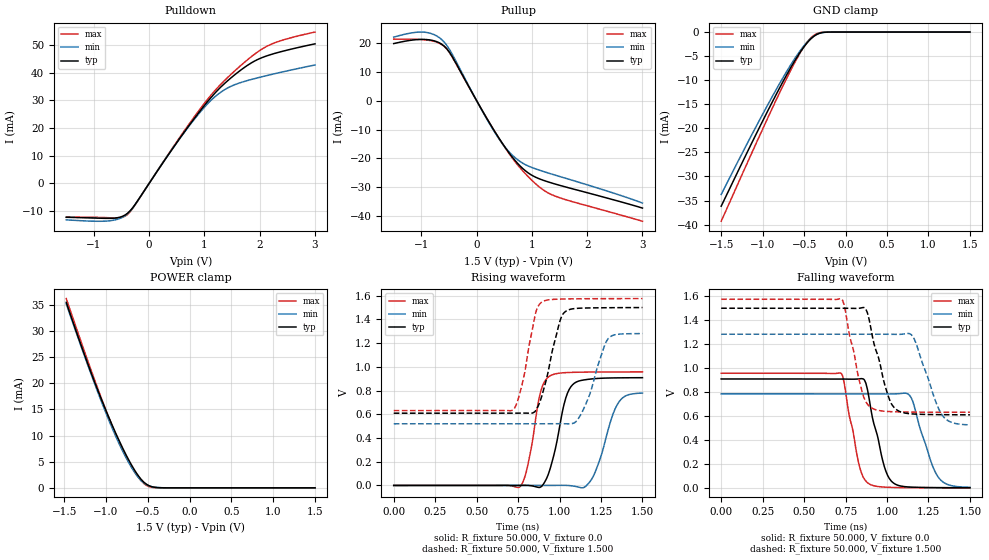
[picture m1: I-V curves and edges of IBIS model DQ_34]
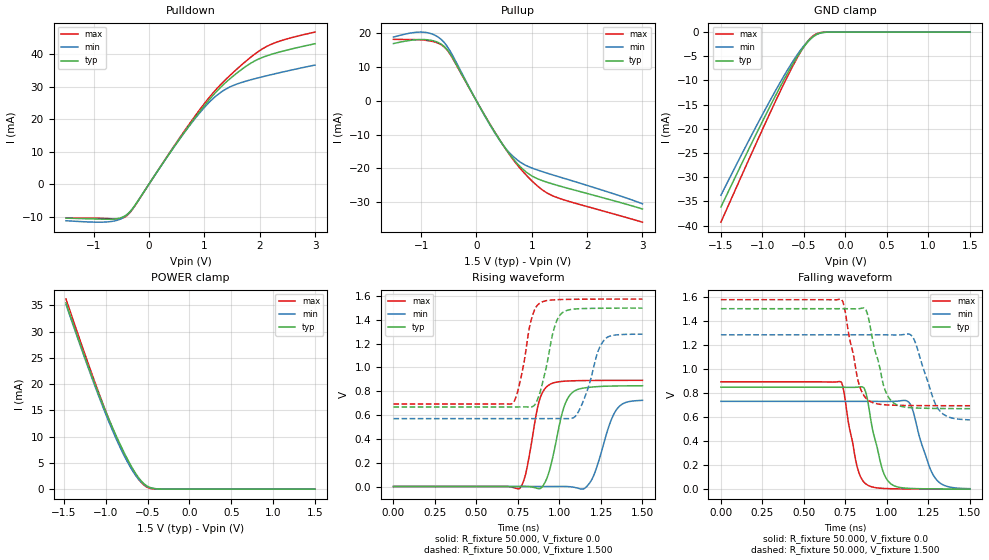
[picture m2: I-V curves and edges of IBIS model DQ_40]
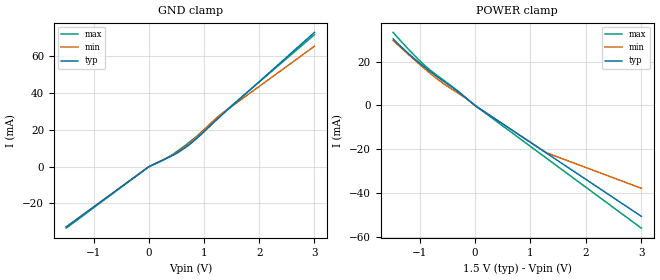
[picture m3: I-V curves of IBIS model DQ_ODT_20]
| This Model is valid for Temperature Range -40C<=Tc<=95C
| Valid for DDR3/DDR3L 1866 operation
| Part Number   VDD   VDDQ   Architecture   Package
| SCB13H8G162EF-11MI   1.35V/1.50V  1.35/1.50v  512Mx16   96-Ball BGA
[IBIS ver] 5.1
[File name] usslh8g16ei.ibs
[File Rev]  1.00
[Date]   2024-09-10
[Source]   Simulation of a silicon level SPICE model
[Notes]
   Date   Revision   Contents
   2024-09-10   1.00   Initial release
[Disclaimer]  The IBIS models are for modeling purpose only and are
   subject to change without any notice. UniIC is not
   responsible for any problems the models may cause.
[Copyright] Copyright 2024 UniIC Semiconductors Corp. All rights reserved
|   Component SCB13H8G162EF-11MI
[Component] SCB13H8G162EF-11MI
[Manufacturer] UniIC Semiconductors Corp.
[Package]
| variable   typ   min   max
R_pkg   1.088   0.726   1.603
L_pkg   2.210nH   1.650nH   4.223nH
C_pkg   1.078pF   0.834pF   1.397pF
[Pin]  signal_name   model_name   R_pin   L_pin   C_pin
A1   VDDQ   Power
A2   DQU5   DQ   1.194   2.482nH   0.989pF
A3   DQU7   DQ   1.212   2.596nH   0.995pF
A7   DQU4   DQ   1.136   2.498nH   0.908pF
A8   VDDQ   Power
A9   VSS   Gnd
B1   VSSQ   Gnd
B2   VDD   Power
B3   VSS   Gnd
B7   DQSUB   DQS   1.034   2.473nH   0.834pF
B8   DQU6   DQ   1.195   2.425nH   0.996pF
B9   VSSQ   Gnd
C1   VDDQ   Power
C2   DQU3   DQ   1.204   2.606nH   0.975pF
C3   DQU1   DQ   1.142   2.378nH   0.906pF
C7   DQSU   DQS   1.04   2.515nH   0.837pF
C8   DQU2   DQ   1.346   2.914nH   1.076pF
C9   VDDQ   Power
D1   VSSQ   Gnd
D2   VDDQ   Power
D3   DMU   DM   1.139   2.526nH   0.869pF
D7   DQU0   DQ   1.212   2.515nH   0.989pF
D8   VSSQ   Gnd
D9   VDD   Power
E1   VSS   Gnd
E2   VSSQ   Gnd
E3   DQL0   DQ   1.088   2.210nH   1.078pF
E7   DML   DM   1.142   2.270nH   1.071pF
E8   VSSQ   Gnd
E9   VDDQ   Power
F1   VDDQ   Power
F2   DQL2   DQ   1.179   2.247nH   1.161pF
F3   DQSL   DQS   0.879   1.897nH   0.875pF
F7   DQL1   DQ   1.107   2.286nH   1.067pF
F8   DQL3   DQ   1.097   2.267nH   1.062pF
F9   VSSQ   Gnd
G1   VSSQ   Gnd
G2   DQL6   DQ   1.169   2.247nH   1.239pF
G3   DQSLB   DQS   0.89   1.927nH   0.867pF
G7   VDD   Power
G8   VSS   Gnd
G9   VSSQ   Gnd
H1   VREFDQ   Power   1.041   2.295nH   1.271pF
H2   VDDQ   Power
H3   DQL4   DQ   1.08   2.278nH   1.098pF
H7   DQL7   DQ   1.107   2.255nH   1.078pF
H8   DQL5   DQ   1.099   2.285nH   1.058pF
H9   VDDQ   Power
J1   NC   NC
J2   VSS   Gnd
J3   RASB   CA   0.965   1.900nH   0.920pF
J7   CK   CK   1.222   2.820nH   1.098pF
J8   VSS   Gnd
J9   NC   NC
K1   ODT   CA   1.603   3.808nH   1.397pF
K2   VDD   Power
K3   CASB   CA   1.118   2.573nH   1.037pF
K7   CKB   CK   1.193   2.809nH   1.078pF
K8   VDD   Power
K9   CKE   CA   1.243   3.102nH   1.097pF
L1   NC   NC
L2   CSB   CA   1.42   3.871nH   1.155pF
L3   WEB   CA   0.976   2.017nH   0.917pF
L7   A10   CA   1.196   2.906nH   1.068pF
L8   ZQ   NC   0.958   2.238nH   1.063pF
L9   NC   NC
M1   VSS   Gnd
M2   BA0   CA   1.28   2.569nH   1.180pF
M3   BA2   CA   1.293   3.106nH   1.079pF
M7   A15   CA   1.351   3.042nH   1.202pF
M8   VREFCA   Power   0.726   1.650nH   0.861pF
M9   VSS   Gnd
N1   VDD   Power
N2   A3   CA   1.238   3.355nH   1.076pF
N3   A0   CA   1.097   3.149nH   0.979pF
N7   A12   CA   1.046   2.533nH   0.972pF
N8   BA1   CA   1.175   2.792nH   1.034pF
N9   VDD   Power
P1   VSS   Gnd
P2   A5   CA   1.211   3.936nH   0.963pF
P3   A2   CA   1.136   3.857nH   0.923pF
P7   A1   CA   1.016   2.953nH   0.869pF
P8   A4   CA   1.022   2.783nH   0.937pF
P9   VSS   Gnd
R1   VDD   Power
R2   A7   CA   1.265   4.223nH   1.016pF
R3   A9   CA   1.243   4.199nH   1.004pF
R7   A11   CA   1.152   3.663nH   0.954pF
R8   A6   CA   1.222   3.809nH   1.017pF
R9   VDD   Power
T1   VSS   Gnd
T2   RESETB   RST   1.573   3.493nH   1.305pF
T3   A13   CA   1.319   3.992nH   1.086pF
T7   A14   CA   1.172   3.553nH   1.018pF
T8   A8   CA   1.124   3.338nH   0.992pF
T9   VSS   Gnd
[Pin Mapping]  pulldown_ref   pullup_ref   gnd_clamp_ref   power_clamp_ref   ext_ref
A1   NC   VDDQ   NC   NC
A2   VSS   VDDQ   VSS   VDDQ
A3   VSS   VDDQ   VSS   VDDQ
A7   VSS   VDDQ   VSS   VDDQ
A8   NC   VDDQ   NC   NC
A9   VSS   NC   NC   NC
B1   VSSQ   NC   NC   NC
B2   NC   VDD   NC   NC
B3   VSS   NC   NC   NC
B7   VSS   VDDQ   VSS   VDDQ
B8   VSS   VDDQ   VSS   VDDQ
B9   VSSQ   NC   NC   NC
C1   NC   VDDQ   NC   NC
C2   VSS   VDDQ   VSS   VDDQ
C3   VSS   VDDQ   VSS   VDDQ
C7   VSS   VDDQ   VSS   VDDQ
C8   VSS   VDDQ   VSS   VDDQ
C9   NC   VDDQ   NC   NC
D1   VSSQ   NC   NC   NC
D2   NC   VDDQ   NC   NC
D3   VSS   VDDQ   VSS   VDDQ
D7   VSS   VDDQ   VSS   VDDQ
D8   VSSQ   NC   NC   NC
D9   NC   VDD   NC   NC
E1   VSS   NC   NC   NC
E2   VSSQ   NC   NC   NC
E3   VSS   VDDQ   VSS   VDDQ
E7   VSS   VDDQ   VSS   VDDQ
E8   VSSQ   NC   NC   NC
E9   NC   VDDQ   NC   NC
F1   NC   VDDQ   NC   NC
F2   VSS   VDDQ   VSS   VDDQ
F3   VSS   VDDQ   VSS   VDDQ
F7   VSS   VDDQ   VSS   VDDQ
F8   VSS   VDDQ   VSS   VDDQ
F9   VSSQ   NC   NC   NC
G1   VSSQ   NC   NC   NC
G2   VSS   VDDQ   VSS   VDDQ
G3   VSS   VDDQ   VSS   VDDQ
G7   NC   VDD   NC   NC
G8   VSS   NC   NC   NC
G9   VSSQ   NC   NC   NC
H1   NC   VREFDQ   NC   NC
H2   NC   VDDQ   NC   NC
H3   VSS   VDDQ   VSS   VDDQ
H7   VSS   VDDQ   VSS   VDDQ
H8   VSS   VDDQ   VSS   VDDQ
H9   NC   VDDQ   NC   NC
J1   NC   NC   NC   NC
J2   VSS   NC   NC   NC
J3   NC   NC   VSS   VDD
J7   NC   NC   VSS   VDD
J8   VSS   NC   NC   NC
J9   NC   NC   NC   NC
K1   NC   NC   VSS   VDD
K2   NC   VDD   NC   NC
K3   NC   NC   VSS   VDD
K7   NC   NC   VSS   VDD
K8   NC   VDD   NC   NC
K9   NC   NC   VSS   VDD
L1   NC   NC   NC   NC
L2   NC   NC   VSS   VDD
L3   NC   NC   VSS   VDD
L7   NC   NC   VSS   VDD
L8   NC   NC   NC   NC
L9   NC   NC   NC   NC
M1   VSS   NC   NC   NC
M2   NC   NC   VSS   VDD
M3   NC   NC   VSS   VDD
M7   NC   NC   VSS   VDD
M8   NC   VREFCA   NC   NC
M9   VSS   NC   NC   NC
N1   NC   VDD   NC   NC
N2   NC   NC   VSS   VDD
N3   NC   NC   VSS   VDD
N7   NC   NC   VSS   VDD
N8   NC   NC   VSS   VDD
N9   NC   VDD   NC   NC
P1   VSS   NC   NC   NC
P2   NC   NC   VSS   VDD
P3   NC   NC   VSS   VDD
P7   NC   NC   VSS   VDD
P8   NC   NC   VSS   VDD
P9   VSS   NC   NC   NC
R1   NC   VDD   NC   NC
R2   NC   NC   VSS   VDD
R3   NC   NC   VSS   VDD
R7   NC   NC   VSS   VDD
R8   NC   NC   VSS   VDD
R9   NC   VDD   NC   NC
T1   VSS   NC   NC   NC
T2   NC   NC   VSS   VDD
T3   NC   NC   VSS   VDD
T7   NC   NC   VSS   VDD
T8   NC   NC   VSS   VDD
T9   VSS   NC   NC   NC
[Diff pin]  inv_pin  vdiff   tdelay_typ   tdelay_min   tdelay_max
J7   K7   0.35   NA   NA   0
C7   B7   0.35   NA   NA   0
F3   G3   0.35   NA   NA   0
[Model Selector] DQ
DQ_34 34 Ohm Data I/O with no ODT
DQ_40 40 Ohm Data I/O with no ODT
DQ_ODT_20 Data Input with 20 Ohm ODT
DQ_ODT_30 Data Input with 30 Ohm ODT
DQ_ODT_40 Data Input with 40 Ohm ODT
DQ_ODT_60 Data Input with 60 Ohm ODT
DQ_ODT_120 Data Input with 120 Ohm ODT
[Model Selector] DQS
DQS_34 34 Ohm Data I/O with no ODT
DQS_40 40 Ohm Data I/O with no ODT
DQS_ODT_20 Data Strobe Input with 20 Ohm ODT
DQS_ODT_30 Data Strobe Input with 30 Ohm ODT
DQS_ODT_40 Data Strobe Input with 40 Ohm ODT
DQS_ODT_60 Data Strobe Input with 60 Ohm ODT
DQS_ODT_120 Data Strobe Input with 120 Ohm ODT
[Model Selector] DM
DQ_34 34 Ohm Data I/O with no ODT
DQ_40 40 Ohm Data I/O with no ODT
DQ_ODT_20 Data Input with 20 Ohm ODT
DQ_ODT_30 Data Input with 30 Ohm ODT
DQ_ODT_40 Data Input with 40 Ohm ODT
DQ_ODT_60 Data Input with 60 Ohm ODT
DQ_ODT_120 Data Input with 120 Ohm ODT
| Models and submodels in the file (17): DQ_34 (I/O), DQ_40 (I/O), DQ_ODT_20 (Input), DQ_ODT_30 (Input), DQ_ODT_40 (Input), DQ_ODT_60 (Input), DQ_ODT_120 (Input), DQS_34 (I/O), DQS_40 (I/O), DQS_ODT_20 (Input), DQS_ODT_30 (Input), DQS_ODT_40 (Input), DQS_ODT_60 (Input), DQS_ODT_120 (Input), CA (Input), CK (Input), RST (Input)
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|   Model DQ_34
[Model] DQ_34
Model_type I/O
Polarity   Non-Inverting
Enable   Active-High
Vinl =  0.615V
Vinh =  0.885V
Vmeas =  0.750V
Rref =  25.000
Vref =  0.750V
C_comp   0.989pF   0.937pF   1.002pF
C_comp_pullup   0.649pF   0.594pF   0.657pF
C_comp_pulldown   0.344pF   0.340pF   0.345pF
[Model Spec]
Vinh   0.885V   0.776V   0.922V
Vinl   0.615V   0.506V   0.652V
Vmeas   0.750V   0.641V   0.787V
Vref   0.750V   0.641V   0.787V
Rref   25.000   25.000   25.000
[Temperature Range]   45.000   95.000   -40.000
[Voltage Range]   1.500V   1.283V   1.575V
[C Comp Corner]
C_comp_pullup   0.657pF   0.594pF   0.649pF
C_comp_pulldown   0.345pF   0.344pF   0.340pF
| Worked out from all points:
|   slope of the pulldown table from 0 to 0.225 V, typ, clamps not added: 33.4 ohm
|   slope of the pullup table from 0 to 0.225 V, typ, clamps not added: 30.2 ohm
|   GND clamp passes 1 mA (typ) near -0.39 V on its own axis
|   POWER clamp passes 1 mA (typ) near -0.54 V on its own axis
|   rising waveform, R_fixture 50.000, V_fixture 0.0: 20-80 % time 84ps typ, 102ps min, 70.1ps max; typ from 0 V to 0.908 V
|   rising waveform, R_fixture 50.000, V_fixture 1.500: 20-80 % time 90.4ps typ, 105ps min, 77.3ps max; typ from 0.609 V to 1.5 V
|   falling waveform, R_fixture 50.000, V_fixture 0.0: 20-80 % time 88.6ps typ, 107ps min, 77.8ps max; typ from 0.909 V to 0.001 V
|   falling waveform, R_fixture 50.000, V_fixture 1.500: 20-80 % time 98.5ps typ, 113ps min, 86.9ps max; typ from 1.5 V to 0.61 V
[Pulldown]
|Voltage   I(typ)   I(min)   I(max)
-1.5V     -12.3mA    -13.23mA   -12.25mA
-718mV    -12.68mA   -13.57mA   -12.47mA
-534mV    -12.28mA   -12.74mA   -12.5mA
-396mV    -10.91mA   -11.08mA   -11.33mA
-258mV    -7.75mA    -7.81mA    -7.928mA
662mV     19.29mA    19.16mA    19.76mA
984mV     27.81mA    27.2mA     28.56mA
1.214V    33.18mA    31.75mA    34.12mA
1.674V    41.24mA    36.59mA    42.95mA
2.088V    45.86mA    38.81mA    49.17mA
2.41V     47.79mA    40.32mA    51.82mA
3V        50.5mA     42.84mA    54.76mA
[Pullup]
|Voltage   I(typ)   I(min)   I(max)
-1.5V     19.78mA    22.01mA    21.32mA
-956mV    21.22mA    23.74mA    21.11mA
-772mV    20.75mA    22.9mA     20.57mA
-588mV    18.92mA    20.32mA    18.82mA
-450mV    15.53mA    16.38mA    15.38mA
148mV     -4.96mA    -5.153mA   -4.926mA
470mV     -14.9mA    -14.99mA   -14.99mA
654mV     -19.76mA   -19.02mA   -20.09mA
838mV     -23.56mA   -21.7mA    -24.38mA
1.16V     -27.25mA   -24.21mA   -30.27mA
1.528V    -29.45mA   -26.4mA    -33.78mA
3V        -37.19mA   -35.46mA   -41.76mA
[GND_clamp]
|Voltage   I(typ)   I(min)   I(max)
-1.5V     -36.19mA   -33.76mA   -39.32mA
-1.066V   -20.77mA   -19.21mA   -22.66mA
-880mV    -14.41mA   -13.29mA   -15.7mA
-725mV    -9.363mA   -8.618mA   -10.11mA
-601mV    -5.649mA   -5.206mA   -5.957mA
-508mV    -3.226mA   -2.993mA   -3.205mA
-446mV    -1.897mA   -1.781mA   -1.722mA
-384mV    -901.4uA   -865.9uA   -696.2uA
-291mV    -146.4uA   -155.4uA   -72.34uA
-198mV    -7.512uA   -11.26uA   -1.231uA
1.5V      0A         0A         0A
[POWER_clamp]
|Voltage   I(typ)   I(min)   I(max)
-1.476V   35.46mA    35.16mA    36.18mA
-1.321V   28.28mA    28.05mA    28.95mA
-1.166V   21.46mA    21.17mA    21.92mA
-1.042V   16.37mA    15.95mA    16.55mA
-918mV    11.66mA    11.09mA    11.53mA
-794mV    7.371mA    6.793mA    7.041mA
-701mV    4.524mA    4.045mA    4.179mA
-608mV    2.178mA    1.886mA    1.878mA
-546mV    1.057mA    913.8uA    793uA
-453mV    217.8uA    210.4uA    93.91uA
-360mV    28.82uA    35.6uA     5.575uA
1.5V      0A         0A         0A
[Ramp]
| variable   typ   min   max
dV/dt_r   0.545/84.699p   0.467/0.102n   0.574/70.583p
dV/dt_f   0.534/98.035p   0.454/0.115n   0.566/87.057p
R_load = 50.000
[Rising Waveform]
R_fixture= 50.000
V_fixture= 0.0
V_fixture_min= 0.0
V_fixture_max= 0.0
|time   V(typ)   V(min)   V(max)
0s        737.6nV    1.747uV    141.1nV
759ps     462.8uV    155.3uV    -14.93mV
807ps     477.5uV    183uV      161.3mV
885ps     -13.67mV   123.7uV    785.7mV
947ps     159.5mV    199.3uV    927mV
1.048ns   779.1mV    -17.91uV   951.8mV
1.146ns   889.2mV    -17.46mV   955.1mV
1.215ns   900.5mV    113.7mV    956mV
1.349ns   906.8mV    683.7mV    956.8mV
1.5ns     908.3mV    778.9mV    957mV
[Rising Waveform]
R_fixture= 50.000
V_fixture= 1.500
V_fixture_min= 1.283
V_fixture_max= 1.575
|time   V(typ)   V(min)   V(max)
0s        609mV      519.8mV    631mV
719ps     609.2mV    519.9mV    635.2mV
772ps     609.7mV    520mV      839mV
840ps     611.8mV    520mV      1.344V
889ps     736mV      519.9mV    1.542V
1.009ns   1.413V     520.3mV    1.571V
1.087ns   1.49V      526.2mV    1.573V
1.174ns   1.496V     738.7mV    1.574V
1.294ns   1.498V     1.239V     1.575V
1.5ns     1.499V     1.28V      1.575V
[Falling Waveform]
R_fixture= 50.000
V_fixture= 0.0
V_fixture_min= 0.0
V_fixture_max= 0.0
|time   V(typ)   V(min)   V(max)
0s        909.2mV    785.1mV    957.1mV
723ps     908.6mV    784.7mV    957.7mV
828ps     909.7mV    784.7mV    212.8mV
858ps     908.7mV    784.7mV    85.99mV
994ps     135.6mV    784.1mV    5.604mV
1.04ns    39.2mV     784.5mV    3.459mV
1.125ns   7.984mV    785.3mV    1.663mV
1.155ns   5.781mV    723.1mV    1.314mV
1.304ns   2.119mV    99.51mV    457.8uV
1.5ns     756.2uV    4.492mV    159uV
[Falling Waveform]
R_fixture= 50.000
V_fixture= 1.500
V_fixture_min= 1.283
V_fixture_max= 1.575
|time   V(typ)   V(min)   V(max)
0s        1.5V       1.283V     1.575V
723ps     1.5V       1.283V     1.58V
741ps     1.5V       1.283V     1.531V
823ps     1.499V     1.283V     955.7mV
864ps     1.504V     1.283V     743.4mV
1.016ns   733.5mV    1.282V     637mV
1.134ns   619.8mV    1.288V     633mV
1.174ns   615.8mV    1.21V      632.4mV
1.334ns   611.2mV    604.1mV    631.5mV
1.5ns     609.9mV    525.6mV    631.2mV
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|   Model DQ_40
[Model] DQ_40
Model_type I/O
Polarity   Non-Inverting
Enable   Active-High
Vinl =  0.615V
Vinh =  0.885V
Vmeas =  0.750V
Rref =  25.000
Vref =  0.750V
C_comp   1.009pF   0.968pF   1.021pF
C_comp_pullup   0.661pF   0.619pF   0.670pF
C_comp_pulldown   0.349pF   0.347pF   0.351pF
[Model Spec]
Vinh   0.885V   0.776V   0.922V
Vinl   0.615V   0.506V   0.652V
Vmeas   0.750V   0.641V   0.787V
Vref   0.750V   0.641V   0.787V
Rref   25.000   25.000   25.000
[Temperature Range]   45.000   95.000   -40.000
[Voltage Range]   1.500V   1.283V   1.575V
[C Comp Corner]
C_comp_pullup   0.670pF   0.619pF   0.661pF
C_comp_pulldown   0.351pF   0.349pF   0.347pF
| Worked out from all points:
|   slope of the pulldown table from 0 to 0.225 V, typ, clamps not added: 39 ohm
|   slope of the pullup table from 0 to 0.225 V, typ, clamps not added: 35.1 ohm
|   GND clamp passes 1 mA (typ) near -0.39 V on its own axis
|   POWER clamp passes 1 mA (typ) near -0.54 V on its own axis
|   rising waveform, R_fixture 50.000, V_fixture 0.0: 20-80 % time 83ps typ, 97.7ps min, 69.3ps max; typ from 0 V to 0.846 V
|   rising waveform, R_fixture 50.000, V_fixture 1.500: 20-80 % time 77.4ps typ, 91.2ps min, 69.2ps max; typ from 0.668 V to 1.5 V
|   falling waveform, R_fixture 50.000, V_fixture 0.0: 20-80 % time 80.2ps typ, 97.4ps min, 70.6ps max; typ from 0.848 V to 0.001 V
|   falling waveform, R_fixture 50.000, V_fixture 1.500: 20-80 % time 84.3ps typ, 99.9ps min, 75.1ps max; typ from 1.5 V to 0.669 V
[Pulldown]
|Voltage   I(typ)   I(min)   I(max)
-1.5V     -10.47mA   -11.25mA   -10.41mA
-718mV    -10.8mA    -11.56mA   -10.62mA
-534mV    -10.48mA   -10.87mA   -10.65mA
-396mV    -9.313mA   -9.46mA    -9.664mA
-258mV    -6.621mA   -6.675mA   -6.77mA
708mV     17.57mA    17.43mA    17.99mA
984mV     23.77mA    23.26mA    24.39mA
1.214V    28.37mA    27.14mA    29.14mA
1.674V    35.27mA    31.27mA    36.68mA
2.088V    39.21mA    33.17mA    41.98mA
2.41V     40.86mA    34.46mA    44.24mA
3V        43.17mA    36.61mA    46.75mA
[Pullup]
|Voltage   I(typ)   I(min)   I(max)
-1.5V     17.01mA    18.93mA    18.26mA
-956mV    18.2mA     20.38mA    18.03mA
-772mV    17.79mA    19.65mA    17.55mA
-588mV    16.23mA    17.43mA    16.08mA
-450mV    13.33mA    14.06mA    13.15mA
194mV     -5.546mA   -5.745mA   -5.5mA
516mV     -13.91mA   -13.87mA   -13.99mA
838mV     -20.27mA   -18.65mA   -20.93mA
1.022V    -22.45mA   -20.04mA   -24.05mA
1.206V    -23.75mA   -21.07mA   -26.59mA
1.574V    -25.59mA   -22.94mA   -29.33mA
3V        -32.07mA   -30.53mA   -35.99mA
[GND_clamp]
|Voltage   I(typ)   I(min)   I(max)
-1.5V     -36.19mA   -33.76mA   -39.32mA
-1.066V   -20.77mA   -19.21mA   -22.66mA
-880mV    -14.41mA   -13.29mA   -15.7mA
-725mV    -9.363mA   -8.618mA   -10.11mA
-601mV    -5.649mA   -5.206mA   -5.957mA
-508mV    -3.226mA   -2.993mA   -3.205mA
-446mV    -1.897mA   -1.781mA   -1.722mA
-384mV    -901.4uA   -865.9uA   -696.2uA
-291mV    -146.4uA   -155.4uA   -72.34uA
-198mV    -7.512uA   -11.26uA   -1.231uA
1.5V      0A         0A         0A
[POWER_clamp]
|Voltage   I(typ)   I(min)   I(max)
-1.476V   35.46mA    35.16mA    36.18mA
-1.321V   28.28mA    28.05mA    28.95mA
-1.166V   21.46mA    21.17mA    21.92mA
-1.042V   16.37mA    15.95mA    16.55mA
-918mV    11.66mA    11.09mA    11.53mA
-794mV    7.371mA    6.793mA    7.041mA
-701mV    4.524mA    4.045mA    4.179mA
-608mV    2.178mA    1.886mA    1.878mA
-546mV    1.057mA    913.8uA    793uA
-453mV    217.8uA    210.4uA    93.91uA
-360mV    28.82uA    35.6uA     5.575uA
1.5V      0A         0A         0A
[Ramp]
| variable   typ   min   max
dV/dt_r   0.508/84.324p   0.434/99.318p   0.535/69.976p
dV/dt_f   0.499/84.534p   0.424/0.103n   0.529/75.094p
R_load = 50.000
[Rising Waveform]
R_fixture= 50.000
V_fixture= 0.0
V_fixture_min= 0.0
V_fixture_max= 0.0
|time   V(typ)   V(min)   V(max)
0s        786nV      1.889uV    135.1nV
760ps     330.3uV    105.6uV    -16.46mV
797ps     753.5uV    112.8uV    108.2mV
883ps     -17.55mV   66.45uV    740.1mV
933ps     102.6mV    52.74uV    849.8mV
1.04ns    713.7mV    345.1uV    885.8mV
1.145ns   827.2mV    -20.32mV   890.1mV
1.204ns   836.5mV    84.66mV    891mV
1.344ns   844.8mV    647.1mV    891.9mV
1.5ns     846.5mV    724mV      892.2mV
[Rising Waveform]
R_fixture= 50.000
V_fixture= 1.500
V_fixture_min= 1.283
V_fixture_max= 1.575
|time   V(typ)   V(min)   V(max)
0s        668.2mV    570.5mV    693.3mV
713ps     668.3mV    570.6mV    694.9mV
760ps     668.6mV    570.6mV    865.2mV
843ps     675.4mV    570.6mV    1.459V
885ps     800.6mV    570.6mV    1.544V
980ps     1.379V     570.9mV    1.569V
1.076ns   1.489V     573.7mV    1.573V
1.135ns   1.495V     689.5mV    1.574V
1.273ns   1.498V     1.237V     1.575V
1.5ns     1.499V     1.28V      1.575V
[Falling Waveform]
R_fixture= 50.000
V_fixture= 0.0
V_fixture_min= 0.0
V_fixture_max= 0.0
|time   V(typ)   V(min)   V(max)
0s        847.6mV    730.1mV    892.5mV
723ps     847.1mV    729.8mV    892.2mV
820ps     847.6mV    729.8mV    189.7mV
859ps     844.8mV    729.8mV    62.86mV
985ps     118.4mV    729mV      5.961mV
1.122ns   7.734mV    732.9mV    1.668mV
1.152ns   5.727mV    672.5mV    1.319mV
1.211ns   3.645mV    367.7mV    850.1uV
1.292ns   2.237mV    90.02mV    488.4uV
1.5ns     751.8uV    4.26mV     158.7uV
[Falling Waveform]
R_fixture= 50.000
V_fixture= 1.500
V_fixture_min= 1.283
V_fixture_max= 1.575
|time   V(typ)   V(min)   V(max)
0s        1.5V       1.283V     1.575V
725ps     1.5V       1.283V     1.579V
744ps     1.5V       1.283V     1.511V
827ps     1.499V     1.283V     895.9mV
864ps     1.505V     1.283V     773mV
998ps     793.6mV    1.283V     700.5mV
1.132ns   678.6mV    1.29V      695.3mV
1.172ns   675mV      1.215V     694.7mV
1.311ns   670.8mV    663.5mV    693.8mV
1.5ns     669.1mV    576.1mV    693.5mV
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|   Model DQ_ODT_20
[Model] DQ_ODT_20
Model_type Input
Polarity   Non-Inverting
Enable   Active-High
Vinl =  0.615V
Vinh =  0.885V
C_comp   0.913pF   0.802pF   0.924pF
C_comp_power_clamp   0.588pF   0.463pF   0.591pF
C_comp_gnd_clamp   0.336pF   0.322pF   0.338pF
[Model Spec]
Vinh   0.885V   0.776V   0.922V
Vinl   0.615V   0.506V   0.652V
[Temperature Range]   45.000   95.000   -40.000
[Voltage Range]   1.500V   1.283V   1.575V
[C Comp Corner]
C_comp_power_clamp   0.588pF   0.463pF   0.591pF
C_comp_gnd_clamp   0.336pF   0.338pF   0.322pF
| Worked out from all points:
|   GND clamp passes 1 mA (typ) near -0.05 V on its own axis
|   POWER clamp passes 1 mA (typ) near -0.05 V on its own axis
[GND_clamp]
|Voltage   I(typ)   I(min)   I(max)
-1.5V     -32.93mA   -32.78mA   -33.5mA
-12mV     -263.4uA   -262.2uA   -268uA
360mV     5.041mA    5.287mA    5.331mA
546mV     8.056mA    8.549mA    9.076mA
732mV     11.94mA    12.66mA    13.28mA
918mV     16.72mA    17.71mA    17.88mA
1.29V     27.25mA    28.19mA    27.83mA
3V        73.09mA    65.56mA    71.82mA
[POWER_clamp]
|Voltage   I(typ)   I(min)   I(max)
-1.476V   30.34mA    29.64mA    33.3mA
-1.104V   21.55mA    21.08mA    23.1mA
-825mV    15.86mA    15.01mA    16.48mA
-608mV    11.77mA    10.71mA    12.3mA
-360mV    7.337mA    6.536mA    7.618mA
12mV      -201.9uA   -200.8uA   -223.5uA
1.283V    -21.59mA   -21.47mA   -23.89mA
3V        -50.48mA   -37.72mA   -55.87mA
